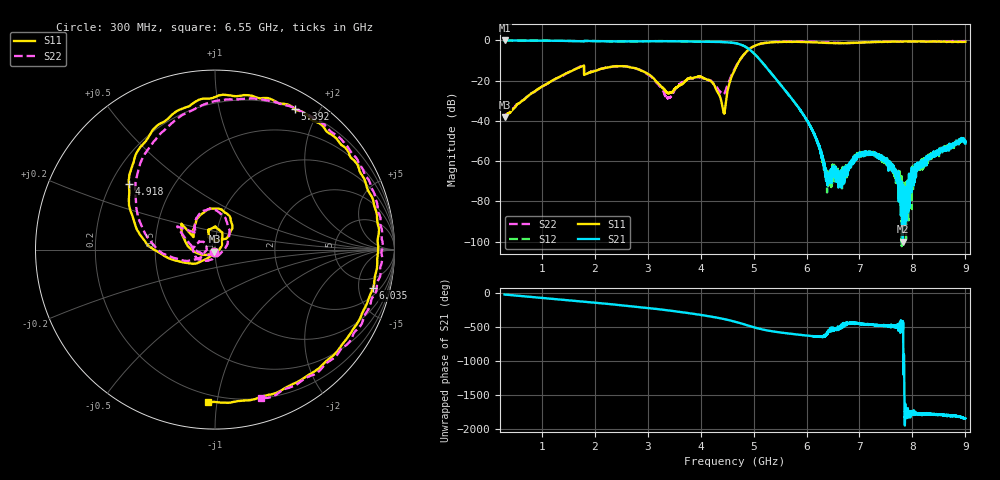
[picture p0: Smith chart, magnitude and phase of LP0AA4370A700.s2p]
!Agilent Technologies,E8358A,US41080443,A.07.50.56
!Agilent E8358A: A.07.50.56
!Date: Monday, December 14, 2015 10:34:19
!Correction: S11(Full 2 Port(1,2))
!S21(Full 2 Port(1,2))
!S12(Full 2 Port(1,2))
!S22(Full 2 Port(1,2))
!S2P File: Measurements: S11, S21, S12, S22:
# Hz S  dB  R 50
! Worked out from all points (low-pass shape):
!   6401 points, 300 MHz to 9 GHz, reference 50 ohm
!   highest |S21| = -0.06 dB at 302.7 MHz (marker M1); lowest = -99.9 dB at 7.82 GHz (marker M2)
!   |S21| within 3 dB of the highest: start of sweep to 4.839 GHz
!   lowest |S11| = -38.1 dB at 300 MHz (marker M3), VSWR 1.03, Z = 49.7 - j1.21 ohm
!   |S11| at or under -10 dB: start of sweep to 4.737 GHz
!   |S22| runs from -38.0 to -0.3 dB; largest |S21 - S12| = 0.015
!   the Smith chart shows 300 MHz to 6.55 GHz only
!   S11 on the Smith chart (normalised r, x): 300 MHz: 0.99, -0.02; 4.918 GHz: 0.27, +0.32; 5.392 GHz: 0.21, +1.70; 6.035 GHz: 2.99, -7.15; 6.55 GHz: 0.15, -0.94
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3e8  -38.05 -103.9  -0.06 -20.4  -0.05 -20.3  -37.98 -104.5
3.027188e8  -37.93 -104.3  -0.06 -20.6  -0.05 -20.5  -37.80 -105.0
1.073484e9  -21.91 -159.5  -0.17 -73.4  -0.15 -73.1  -22.05 -165.5
1.750453e9  -13.05 147.3  -0.43 -120.8  -0.40 -120.4  -12.71 150.8
2.508984e9  -12.83 87.9  -0.53 -177.4  -0.51 -177.0  -12.84 98.6
3.200906e9  -21.35 45.2  -0.38 124.7  -0.36 125.4  -21.88 28.3
3.400734e9  -26.09 83.8  -0.41 105.6  -0.38 106.1  -28.46 -56.9
3.818062e9  -18.64 106.3  -0.60 62.1  -0.53 62.6  -18.78 -161.0
4.201406e9  -20.41 64.3  -0.73 15.3  -0.68 15.8  -20.11 152.4
4.436578e9  -35.91 -41.6  -0.87 -19.5  -0.83 -18.8  -26.74 -179.2
4.65e9  -14.30 -158.6  -1.39 -58.7  -1.31 -58.1  -13.91 -163.8
4.917797e9  -4.37 142.7  -4.44 -120.5  -4.41 -120.2  -4.40 135.9
5.392219e9  -0.91 60.3  -18.25 155.1  -18.18 156.0  -0.75 52.6
6.035203e9  -0.85 -13.6  -41.04 94.2  -40.99 95.8  -0.61 -3.8
6.100453e9  -0.97 -21.8  -44.22 87.9  -44.00 89.6  -0.65 -10.2
6.394078e9  -1.23 -65.7  -72.02 135.9  -67.72 134.7  -1.06 -46.4
6.550406e9  -1.39 -93.1  -65.86 -160.1  -66.64 176.3  -1.27 -73.1
7.001719e9  -1.10 -165.6  -55.75 -91.0  -56.73 -83.5  -1.08 -154.0
7.550906e9  -0.67 149.2  -61.01 -108.7  -59.88 -116.1  -0.58 151.4
7.820062e9  -0.63 138.2  -99.93 -49.7  -70.62 -104.0  -0.48 134.1
8.127281e9  -0.54 126.2  -61.79 31.8  -61.29 25.3  -0.46 118.7
9e9  -0.64 96.4  -51.24 -39.3  -50.91 -27.5  -0.38 66.5
